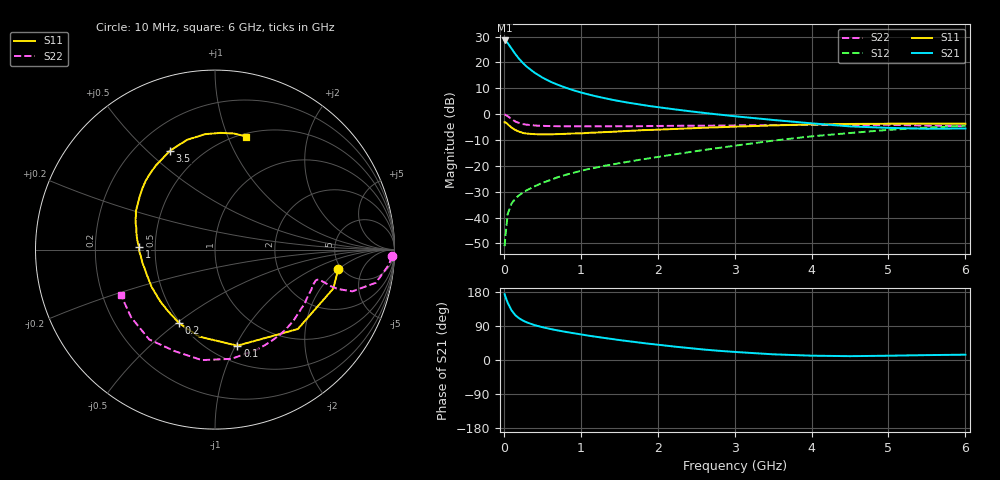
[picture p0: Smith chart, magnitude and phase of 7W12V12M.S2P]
! Infineon Technologies  Discrete & RF Semiconductors
! BFS17W
! Si NPN RF Bipolar Junction Transistor in SOT323
! VCE = 12 V  IC = 12 mA
! Common Emitter S-Parameters:  August  1999
# GHz  S  MA  R  50
!  f  S11  S21  S12  S22
! GHz  MAG  ANG  MAG  ANG  MAG  ANG  MAG  ANG
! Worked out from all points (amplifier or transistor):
!   36 points, 10 MHz to 6 GHz, reference 50 ohm
!   highest |S21| = 28.5 dB at 10 MHz (marker M1)
!   |S21| within 3 dB of that: start of sweep to 96.85 MHz
!   unconditionally stable (mu >= 1): 421 MHz to 2.058 GHz; 5.767 GHz to end of sweep
!   at 250 MHz: K = 0.80, MSG = 25.0 dB, |S12| = -30.3 dB
!   at 1.4 GHz: K = 1.14, MAG = 10.3 dB, |S12| = -19.5 dB
!   at 6 GHz: K = 1.02, MAG = -1.3 dB, |S12| = -4.5 dB
!   S11 on the Smith chart (normalised r, x): 10 MHz: 4.68, -1.99; 100 MHz: 0.66, -1.02; 200 MHz: 0.49, -0.51; 1 GHz: 0.40, +0.01; 3.5 GHz: 0.34, +0.59; 6 GHz: 0.53, +1.16
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0.01  0.6952 -9.1  26.54 173.6  0.0028 77.8  0.9885 -2.2
0.02  0.6936 -18.3  26.13 167.3  0.0043 83.3  0.9713 -5.1
0.05  0.6393 -43.8  23.68 150.9  0.0117 73.3  0.9158 -11.6
0.1  0.5496 -76.9  18.5 131.1  0.0186 61.0  0.7998 -16.9
0.15  0.4927 -100.4  14.46 118.2  0.0234 56.6  0.7184 -17.8
0.2  0.4563 -115.9  11.66 109.9  0.0271 57.3  0.6711 -17.5
0.25  0.4312 -127.5  9.648 103.9  0.0306 57.6  0.6416 -16.8
0.3  0.4201 -136.5  8.209 99.2  0.0338 58.9  0.6244 -16.5
0.4  0.4099 -149.5  6.309 92.0  0.0401 61.4  0.6028 -16.2
0.5  0.4049 -158.2  5.105 86.7  0.047 63.5  0.5934 -16.4
0.6  0.4062 -164.8  4.277 82.1  0.0528 65.8  0.5871 -17.1
0.7  0.4109 -170.0  3.698 78.1  0.0603 66.9  0.5839 -18.3
0.8  0.4153 -174.9  3.255 74.3  0.0668 67.7  0.581 -19.6
1  0.4239 178.0  2.625 67.6  0.0801 69.3  0.5818 -22.4
1.1  0.4341 174.0  2.401 64.2  0.0866 69.7  0.5797 -24.4
1.6  0.4734 159.3  1.679 50.1  0.1189 71.8  0.5822 -34.2
2.2  0.5146 144.4  1.247 35.8  0.1652 74.3  0.5936 -47.8
2.8  0.5579 130.1  0.979 24.2  0.2226 74.0  0.6009 -62.8
3.5  0.6056 114.4  0.771 15.0  0.3071 70.4  0.6156 -81.4
4.5  0.6455 95.0  0.579 10.1  0.4312 58.9  0.6087 -111.7
5.5  0.6557 80.5  0.521 12.9  0.5479 45.6  0.6004 -141.1
6  0.6528 74.8  0.528 14.0  0.5954 38.9  0.5822 -154.5
